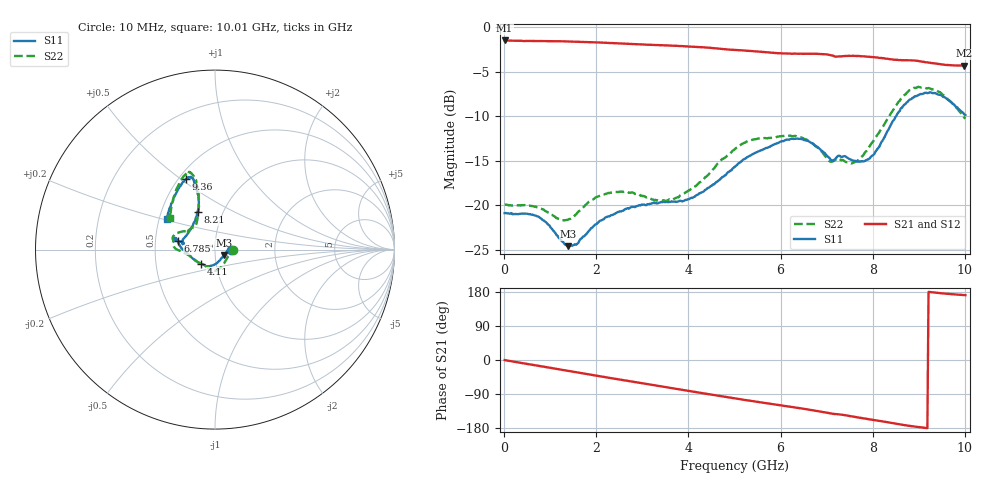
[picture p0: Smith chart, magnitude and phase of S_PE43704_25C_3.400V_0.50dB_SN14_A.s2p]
! Device ID: PE43704
! Dir: z:\PE43704\PE43704_Char_1_20130516\PE43704\AMB\3p400V\0p50dB
! Serial: 14
! Insertion: A
! Impedance: 50 ohm
! Temp: Amb
! VDD: 3.400V
! Attenuation Step: 0.50dB
! IDD: 1.140682e-01mA
#  Hz  S  RI  R  50
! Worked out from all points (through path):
!   401 points, 10 MHz to 10.01 GHz, reference 50 ohm
!   highest |S21| = -1.51 dB at 10 MHz (marker M1); lowest = -4.3 dB at 9.985 GHz (marker M2)
!   group delay of S21, straight-line fit = 53.7 ps
!   lowest |S11| = -24.6 dB at 1.385 GHz (marker M3), VSWR 1.12, Z = 55.1 - j3.45 ohm
!   |S11| at or under -10 dB: start of sweep to 8.51 GHz
!   |S22| runs from -21.7 to -6.7 dB; largest |S21 - S12| = 0.006
!   S11 on the Smith chart (normalised r, x): 10 MHz: 1.20, +0.00; 4.11 GHz: 0.84, -0.13; 6.785 GHz: 0.65, +0.06; 8.21 GHz: 0.76, +0.33; 9.36 GHz: 0.54, +0.52; 10.01 GHz: 0.55, +0.21
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1e7  0.09 0.000161  0.8404 -0.00338  0.8405 -0.00344  0.1005 9.81e-05
7.35e8  0.0848 0.0161  0.8048 -0.2183  0.8047 -0.2181  0.0964 0.0074
1.385e9  0.0498 -0.0312  0.7283 -0.3978  0.7282 -0.3978  0.0659 -0.0499
1.685e9  0.0277 -0.0589  0.6775 -0.4727  0.6775 -0.4726  0.0444 -0.0839
2.41e9  -0.0165 -0.088  0.5245 -0.6183  0.5249 -0.6177  -0.00547 -0.1182
3.36e9  -0.0398 -0.0949  0.2891 -0.7365  0.2897 -0.7361  -0.0452 -0.0958
4.11e9  -0.0791 -0.0775  0.0856 -0.7698  0.0865 -0.7697  -0.1123 -0.0579
5.01e9  -0.1641 -0.0122  -0.1461 -0.7289  -0.1457 -0.7291  -0.2065 -0.00258
5.36e9  -0.1903 0.013  -0.2271 -0.6973  -0.227 -0.6974  -0.2303 0.0204
6.085e9  -0.2209 0.0652  -0.3648 -0.6095  -0.3627 -0.6089  -0.2364 0.0642
6.685e9  -0.2168 0.05  -0.4779 -0.5218  -0.4783 -0.5204  -0.2002 0.096
6.785e9  -0.2074 0.0472  -0.4957 -0.5041  -0.4971 -0.5032  -0.1868 0.1
7.085e9  -0.1757 0.0391  -0.5387 -0.4401  -0.5409 -0.4407  -0.1484 0.0929
7.585e9  -0.1584 0.0792  -0.594 -0.3485  -0.5931 -0.3478  -0.1075 0.136
7.885e9  -0.1298 0.1249  -0.621 -0.2801  -0.6207 -0.2825  -0.097 0.1801
8.21e9  -0.0974 0.2077  -0.6352 -0.2076  -0.6345 -0.2126  -0.0903 0.2571
8.36e9  -0.0902 0.2559  -0.6377 -0.1706  -0.6378 -0.1738  -0.0908 0.3029
8.835e9  -0.1154 0.3763  -0.6463 -0.0618  -0.6422 -0.064  -0.1316 0.4234
9.36e9  -0.163 0.3924  -0.6233 0.0248  -0.6237 0.0261  -0.1774 0.4052
9.635e9  -0.2091 0.3285  -0.608 0.0588  -0.6079 0.0593  -0.2185 0.3249
9.985e9  -0.2647 0.1848  -0.5999 0.0915  -0.6024 0.094  -0.2492 0.1837
1.001e10  -0.2699 0.1722  -0.6016 0.0939  -0.6054 0.0952  -0.2513 0.1736
